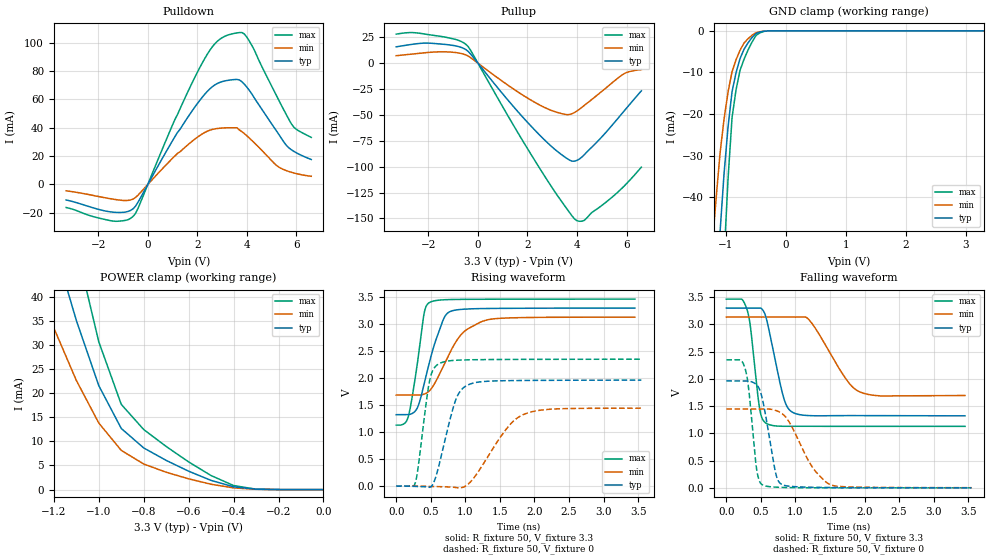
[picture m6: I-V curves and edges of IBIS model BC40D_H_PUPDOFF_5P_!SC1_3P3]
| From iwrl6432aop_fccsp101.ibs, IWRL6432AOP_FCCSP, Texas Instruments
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|   Model Cell BC40D_H_PUPDOFF_5P_!SC1_3P3
|BC40D_H_PUPDOFF_5P_!SC1_3P3
[Model]   BC40D_H_PUPDOFF_5P_!SC1_3P3
Model_type   I/O
Polarity   Non-Inverting
Enable   Active-Low
Vinl =  0.8V
Vinh =  2V
Cref =  15pF
Rref =  100.0000M
Vref =  0V
Vmeas =  1.65
C_comp   2.157014p   1.964007p   2.198404p
|[Input load] weak_pupdoff
|[Output drive] fast
|[supplytol] 5
|[temp] ind
[Model Spec]
Vinl   0.8V   0.8V   0.8V
Vinh   2V   2V   2V
[Temperature Range]   25   125   -40
[Voltage Range]   3.3   3.135   3.465
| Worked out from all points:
|   slope of the pulldown table from 0 to 0.495 V, typ, clamps not added: 31.8 ohm
|   slope of the pullup table from 0 to 0.495 V, typ, clamps not added: 33.3 ohm
|   GND clamp passes 1 mA (typ) near -0.53 V on its own axis
|   POWER clamp passes 1 mA (typ) near -0.43 V on its own axis
|   rising waveform, R_fixture 50, V_fixture 3.3: 20-80 % time 258ps typ, 377ps min, 156ps max; typ from 1.32 V to 3.3 V
|   rising waveform, R_fixture 50, V_fixture 0: 20-80 % time 233ps typ, 458ps min, 142ps max; typ from 0 V to 1.96 V
|   falling waveform, R_fixture 50, V_fixture 3.3: 20-80 % time 199ps typ, 411ps min, 121ps max; typ from 3.3 V to 1.32 V
|   falling waveform, R_fixture 50, V_fixture 0: 20-80 % time 162ps typ, 365ps min, 108ps max; typ from 1.96 V to 0 V
| Nom Voltages:
|   VDD=1.1, VDDS=3.3, VDDS18=1.8, ESD_BIASFET=0, VSS=0, VSSS=0
| Min Voltages:
|   VDD=1.045, VDDS=3.135, VDDS18=1.71, ESD_BIASFET=0, VSS=0, VSSS=0
| Max Voltages:
|   VDD=1.16, VDDS=3.465, VDDS18=1.89, ESD_BIASFET=0, VSS=0, VSSS=0
[POWER_clamp]
|   voltage   I(typ)   I(min)   I(max)
-3.3V     446.9mA    437.1mA    604mA
-1.267V   62.17mA    41.49mA    88.04mA
-1.233V   56.52mA    37.49mA    80.24mA
-1.133V   40.34mA    26.26mA    57.63mA
-1.067V   30.56mA    19.69mA    43.69mA
-1.033V   26.05mA    16.74mA    37.16mA
-1V       21.55mA    13.79mA    30.63mA
-900mV    12.68mA    8.13mA     17.66mA
-800mV    8.63mA     5.305mA    12.44mA
-600mV    3.813mA    2.231mA    5.735mA
-400mV    580.7uA    357.4uA    841.8uA
0V        4.589uA    2.331uA    8.159uA
[Pulldown]
|   voltage   I(typ)   I(min)   I(max)
-3.3V     -10.92mA   -4.469mA   -16.24mA
-1.4V     -19.52mA   -10.37mA   -25.81mA
-600mV    -17.22mA   -10.34mA   -22.6mA
-400mV    -12.67mA   -7.623mA   -17.05mA
1.2V      36.7mA     21.92mA    49.35mA
2.1V      59.3mA     34.49mA    82.4mA
2.7V      70.09mA    39.15mA    99.03mA
3.3V      73.56mA    39.95mA    105.7mA
3.9V      70.66mA    35.84mA    106mA
5.2V      37.64mA    13.39mA    62.46mA
5.8V      24.43mA    8.578mA    42.66mA
6.6V      17.6mA     5.765mA    33.17mA
[Pullup]
|   voltage   I(typ)   I(min)   I(max)
-3.3V     15.77mA    7.22mA     28.03mA
-2.7V     18.05mA    8.673mA    29.54mA
-1.9V     19.23mA    10.53mA    27.2mA
-900mV    16.69mA    10.25mA    22.94mA
-400mV    11.53mA    6.969mA    16.15mA
1.4V      -40.96mA   -24.37mA   -58.54mA
2.6V      -72.01mA   -41.71mA   -105.6mA
3.6V      -92.16mA   -49.74mA   -141mA
4V        -93.88mA   -46.2mA    -152.2mA
4.3V      -88.33mA   -40.72mA   -151.7mA
5.9V      -46.29mA   -10.2mA    -118.8mA
6.6V      -26.71mA   -6.269mA   -100.4mA
[GND_clamp]
|   voltage   I(typ)   I(min)   I(max)
-3.3V     -787.2mA   -627.7mA   -1.235A
-1.233V   -85.66mA   -52.14mA   -138.8mA
-1.167V   -66.47mA   -40.37mA   -107.7mA
-1.1V     -48.25mA   -29.37mA   -77.98mA
-1.033V   -34.27mA   -21.19mA   -54.56mA
-966.7mV  -23.06mA   -14.66mA   -35.5mA
-900mV    -14.61mA   -9.789mA   -20.83mA
-833.3mV  -10.05mA   -6.934mA   -14.15mA
-700mV    -4.416mA   -2.931mA   -6.81mA
-500mV    -621.6uA   -443.6uA   -1.094mA
-300mV    -17.13uA   -24.35uA   -23.51uA
3.3V      4.589uA    5.188uA    6.318uA
[Ramp]
| variable   typ   min   max
dV/dt_f  1.1960322/0.20096998n 0.89007987/0.42414797n  1.4076441/0.12185787n
dV/dt_r  1.1926881/0.2359305n  0.8893036/0.4700993n   1.420701/0.14341063n
R_load = 50
[Rising Waveform]
R_fixture = 50
V_fixture = 3.3
V_fixture_min = 3.135
V_fixture_max = 3.465
|   time   V(typ)   V(min)   V(max)
0s        1.323V     1.686V     1.129V
175.4ps   1.323V     1.686V     1.289V
303ps     1.443V     1.686V     2.245V
403.9ps   1.892V     1.703V     3.201V
488.2ps   2.331V     1.775V     3.407V
666ps     3.036V     2.18V      3.451V
736.9ps   3.198V     2.371V     3.456V
958.1ps   3.276V     2.833V     3.46V
1.258ns   3.29V      3.058V     3.463V
3.453ns   3.299V     3.131V     3.465V
[Rising Waveform]
R_fixture = 50
V_fixture = 0
V_fixture_min = 0
V_fixture_max = 0
|   time   V(typ)   V(min)   V(max)
0s        0V         0V         0V
274.9ps   -6.689mV   0V         52.25mV
480.5ps   -23.36mV   -4.905mV   1.934V
543.2ps   65.04mV    -6.663mV   2.176V
621.2ps   395.5mV    -8.966mV   2.269V
861.3ps   1.596V     -28.02mV   2.331V
1.052ns   1.882V     46.58mV    2.34V
1.589ns   1.953V     1.05V      2.347V
1.843ns   1.957V     1.327V     2.348V
3.547ns   1.963V     1.443V     2.351V
[Falling Waveform]
R_fixture = 50
V_fixture = 3.3
V_fixture_min = 3.135
V_fixture_max = 3.465
|   time   V(typ)   V(min)   V(max)
0s        3.3V       3.134V     3.464V
301ps     3.3V       3.134V     3.266V
351.3ps   3.3V       3.134V     2.93V
482.7ps   3.3V       3.134V     1.449V
583.3ps   3.086V     3.134V     1.18V
827.6ps   1.662V     3.134V     1.13V
969.8ps   1.379V     3.134V     1.13V
1.206ns   1.326V     3.071V     1.13V
1.923ns   1.326V     1.766V     1.129V
3.453ns   1.322V     1.695V     1.129V
[Falling Waveform]
R_fixture = 50
V_fixture = 0
V_fixture_min = 0
V_fixture_max = 0
|   time   V(typ)   V(min)   V(max)
0s        1.963V     1.448V     2.35V
273.2ps   1.963V     1.448V     2.183V
322.1ps   1.96V      1.448V     1.832V
438.8ps   1.889V     1.448V     340mV
527.5ps   1.6V       1.448V     51.23mV
716.6ps   256mV      1.421V     12.97mV
819.3ps   53.32mV    1.35V      7.684mV
1.239ns   10.78mV    391.7mV    0V
1.505ns   6.979mV    59.19mV    0V
3.547ns   0V         3.354mV    0V
